DATA_BLOCK "DB_ASI"
TITLE =
VERSION : 0.1


  STRUCT
   SLAVE_1A_IN1 : BOOL ;
   SLAVE_1A_IN2 : BOOL ;
   SLAVE_1A_IN3 : BOOL ;
   SLAVE_1A_IN4 : BOOL ;
   RISERVATO1 : BOOL ;
   RISERVATO2 : BOOL ;
   RISERVATO3 : BOOL ;
   RISERVATO4 : BOOL ;
   SLAVE_3A_IN1 : BOOL ;
   SLAVE_3A_IN2 : BOOL ;
   SLAVE_3A_IN3 : BOOL ;
   SLAVE_3A_IN4 : BOOL ;
   SLAVE_2A_IN1 : BOOL ;
   SLAVE_2A_IN2 : BOOL ;
   SLAVE_2A_IN3 : BOOL ;
   SLAVE_2A_IN4 : BOOL ;
   SLAVE_5A_IN1 : BOOL ;
   SLAVE_5A_IN2 : BOOL ;
   SLAVE_5A_IN3 : BOOL ;
   SLAVE_5A_IN4 : BOOL ;
   SLAVE_4A_IN1 : BOOL ;
   SLAVE_4A_IN2 : BOOL ;
   SLAVE_4A_IN3 : BOOL ;
   SLAVE_4A_IN4 : BOOL ;
   SLAVE_7A_IN1 : BOOL ;
   SLAVE_7A_IN2 : BOOL ;
   SLAVE_7A_IN3 : BOOL ;
   SLAVE_7A_IN4 : BOOL ;
   SLAVE_6A_IN1 : BOOL ;
   SLAVE_6A_IN2 : BOOL ;
   SLAVE_6A_IN3 : BOOL ;
   SLAVE_6A_IN4 : BOOL ;
   SLAVE_9A_IN1 : BOOL ;
   SLAVE_9A_IN2 : BOOL ;
   SLAVE_9A_IN3 : BOOL ;
   SLAVE_9A_IN4 : BOOL ;
   SLAVE_8A_IN1 : BOOL ;
   SLAVE_8A_IN2 : BOOL ;
   SLAVE_8A_IN3 : BOOL ;
   SLAVE_8A_IN4 : BOOL ;
   SLAVE_11A_IN1 : BOOL ;
   SLAVE_11A_IN2 : BOOL ;
   SLAVE_11A_IN3 : BOOL ;
   SLAVE_11A_IN4 : BOOL ;
   SLAVE_10A_IN1 : BOOL ;
   SLAVE_10A_IN2 : BOOL ;
   SLAVE_10A_IN3 : BOOL ;
   SLAVE_10A_IN4 : BOOL ;
   SLAVE_13A_IN1 : BOOL ;
   SLAVE_13A_IN2 : BOOL ;
   SLAVE_13A_IN3 : BOOL ;
   SLAVE_13A_IN4 : BOOL ;
   SLAVE_12A_IN1 : BOOL ;
   SLAVE_12A_IN2 : BOOL ;
   SLAVE_12A_IN3 : BOOL ;
   SLAVE_12A_IN4 : BOOL ;
   SLAVE_15A_IN1 : BOOL ;
   SLAVE_15A_IN2 : BOOL ;
   SLAVE_15A_IN3 : BOOL ;
   SLAVE_15A_IN4 : BOOL ;
   SLAVE_14A_IN1 : BOOL ;
   SLAVE_14A_IN2 : BOOL ;
   SLAVE_14A_IN3 : BOOL ;
   SLAVE_14A_IN4 : BOOL ;
   SLAVE_17A_IN1 : BOOL ;
   SLAVE_17A_IN2 : BOOL ;
   SLAVE_17A_IN3 : BOOL ;
   SLAVE_17A_IN4 : BOOL ;
   SLAVE_16A_IN1 : BOOL ;
   SLAVE_16A_IN2 : BOOL ;
   SLAVE_16A_IN3 : BOOL ;
   SLAVE_16A_IN4 : BOOL ;
   SLAVE_19A_IN1 : BOOL ;
   SLAVE_19A_IN2 : BOOL ;
   SLAVE_19A_IN3 : BOOL ;
   SLAVE_19A_IN4 : BOOL ;
   SLAVE_18A_IN1 : BOOL ;
   SLAVE_18A_IN2 : BOOL ;
   SLAVE_18A_IN3 : BOOL ;
   SLAVE_18A_IN4 : BOOL ;
   SLAVE_21A_IN1 : BOOL ;
   SLAVE_21A_IN2 : BOOL ;
   SLAVE_21A_IN3 : BOOL ;
   SLAVE_21A_IN4 : BOOL ;
   SLAVE_20A_IN1 : BOOL ;
   SLAVE_20A_IN2 : BOOL ;
   SLAVE_20A_IN3 : BOOL ;
   SLAVE_20A_IN4 : BOOL ;
   SLAVE_23A_IN1 : BOOL ;
   SLAVE_23A_IN2 : BOOL ;
   SLAVE_23A_IN3 : BOOL ;
   SLAVE_23A_IN4 : BOOL ;
   SLAVE_22A_IN1 : BOOL ;
   SLAVE_22A_IN2 : BOOL ;
   SLAVE_22A_IN3 : BOOL ;
   SLAVE_22A_IN4 : BOOL ;
   SLAVE_25A_IN1 : BOOL ;
   SLAVE_25A_IN2 : BOOL ;
   SLAVE_25A_IN3 : BOOL ;
   SLAVE_25A_IN4 : BOOL ;
   SLAVE_24A_IN1 : BOOL ;
   SLAVE_24A_IN2 : BOOL ;
   SLAVE_24A_IN3 : BOOL ;
   SLAVE_24A_IN4 : BOOL ;
   SLAVE_27A_IN1 : BOOL ;
   SLAVE_27A_IN2 : BOOL ;
   SLAVE_27A_IN3 : BOOL ;
   SLAVE_27A_IN4 : BOOL ;
   SLAVE_26A_IN1 : BOOL ;
   SLAVE_26A_IN2 : BOOL ;
   SLAVE_26A_IN3 : BOOL ;
   SLAVE_26A_IN4 : BOOL ;
   SLAVE_29A_IN1 : BOOL ;
   SLAVE_29A_IN2 : BOOL ;
   SLAVE_29A_IN3 : BOOL ;
   SLAVE_29A_IN4 : BOOL ;
   SLAVE_28A_IN1 : BOOL ;
   SLAVE_28A_IN2 : BOOL ;
   SLAVE_28A_IN3 : BOOL ;
   SLAVE_28A_IN4 : BOOL ;
   SLAVE_31A_IN1 : BOOL ;
   SLAVE_31A_IN2 : BOOL ;
   SLAVE_31A_IN3 : BOOL ;
   SLAVE_31A_IN4 : BOOL ;
   SLAVE_30A_IN1 : BOOL ;
   SLAVE_30A_IN2 : BOOL ;
   SLAVE_30A_IN3 : BOOL ;
   SLAVE_30A_IN4 : BOOL ;
   SLAVE_1B_IN1 : BOOL ;
   SLAVE_1B_IN2 : BOOL ;
   SLAVE_1B_IN3 : BOOL ;
   SLAVE_1B_IN4 : BOOL ;
   RISERVATO5 : BOOL ;
   RISERVATO6 : BOOL ;
   RISERVATO7 : BOOL ;
   RISERVATO8 : BOOL ;
   SLAVE_3B_IN1 : BOOL ;
   SLAVE_3B_IN2 : BOOL ;
   SLAVE_3B_IN3 : BOOL ;
   SLAVE_3B_IN4 : BOOL ;
   SLAVE_2B_IN1 : BOOL ;
   SLAVE_2B_IN2 : BOOL ;
   SLAVE_2B_IN3 : BOOL ;
   SLAVE_2B_IN4 : BOOL ;
   SLAVE_5B_IN1 : BOOL ;
   SLAVE_5B_IN2 : BOOL ;
   SLAVE_5B_IN3 : BOOL ;
   SLAVE_5B_IN4 : BOOL ;
   SLAVE_4B_IN1 : BOOL ;
   SLAVE_4B_IN2 : BOOL ;
   SLAVE_4B_IN3 : BOOL ;
   SLAVE_4B_IN4 : BOOL ;
   SLAVE_7B_IN1 : BOOL ;
   SLAVE_7B_IN2 : BOOL ;
   SLAVE_7B_IN3 : BOOL ;
   SLAVE_7B_IN4 : BOOL ;
   SLAVE_6B_IN1 : BOOL ;
   SLAVE_6B_IN2 : BOOL ;
   SLAVE_6B_IN3 : BOOL ;
   SLAVE_6B_IN4 : BOOL ;
   SLAVE_9B_IN1 : BOOL ;
   SLAVE_9B_IN2 : BOOL ;
   SLAVE_9B_IN3 : BOOL ;
   SLAVE_9B_IN4 : BOOL ;
   SLAVE_8B_IN1 : BOOL ;
   SLAVE_8B_IN2 : BOOL ;
   SLAVE_8B_IN3 : BOOL ;
   SLAVE_8B_IN4 : BOOL ;
   SLAVE_11B_IN1 : BOOL ;
   SLAVE_11B_IN2 : BOOL ;
   SLAVE_11B_IN3 : BOOL ;
   SLAVE_11B_IN4 : BOOL ;
   SLAVE_10B_IN1 : BOOL ;
   SLAVE_10B_IN2 : BOOL ;
   SLAVE_10B_IN3 : BOOL ;
   SLAVE_10B_IN4 : BOOL ;
   SLAVE_13B_IN1 : BOOL ;
   SLAVE_13B_IN2 : BOOL ;
   SLAVE_13B_IN3 : BOOL ;
   SLAVE_13B_IN4 : BOOL ;
   SLAVE_12B_IN1 : BOOL ;
   SLAVE_12B_IN2 : BOOL ;
   SLAVE_12B_IN3 : BOOL ;
   SLAVE_12B_IN4 : BOOL ;
   SLAVE_15B_IN1 : BOOL ;
   SLAVE_15B_IN2 : BOOL ;
   SLAVE_15B_IN3 : BOOL ;
   SLAVE_15B_IN4 : BOOL ;
   SLAVE_14B_IN1 : BOOL ;
   SLAVE_14B_IN2 : BOOL ;
   SLAVE_14B_IN3 : BOOL ;
   SLAVE_14B_IN4 : BOOL ;
   SLAVE_17B_IN1 : BOOL ;
   SLAVE_17B_IN2 : BOOL ;
   SLAVE_17B_IN3 : BOOL ;
   SLAVE_17B_IN4 : BOOL ;
   SLAVE_16B_IN1 : BOOL ;
   SLAVE_16B_IN2 : BOOL ;
   SLAVE_16B_IN3 : BOOL ;
   SLAVE_16B_IN4 : BOOL ;
   SLAVE_19B_IN1 : BOOL ;
   SLAVE_19B_IN2 : BOOL ;
   SLAVE_19B_IN3 : BOOL ;
   SLAVE_19B_IN4 : BOOL ;
   SLAVE_18B_IN1 : BOOL ;
   SLAVE_18B_IN2 : BOOL ;
   SLAVE_18B_IN3 : BOOL ;
   SLAVE_18B_IN4 : BOOL ;
   SLAVE_21B_IN1 : BOOL ;
   SLAVE_21B_IN2 : BOOL ;
   SLAVE_21B_IN3 : BOOL ;
   SLAVE_21B_IN4 : BOOL ;
   SLAVE_20B_IN1 : BOOL ;
   SLAVE_20B_IN2 : BOOL ;
   SLAVE_20B_IN3 : BOOL ;
   SLAVE_20B_IN4 : BOOL ;
   SLAVE_23B_IN1 : BOOL ;
   SLAVE_23B_IN2 : BOOL ;
   SLAVE_23B_IN3 : BOOL ;
   SLAVE_23B_IN4 : BOOL ;
   SLAVE_22B_IN1 : BOOL ;
   SLAVE_22B_IN2 : BOOL ;
   SLAVE_22B_IN3 : BOOL ;
   SLAVE_22B_IN4 : BOOL ;
   SLAVE_25B_IN1 : BOOL ;
   SLAVE_25B_IN2 : BOOL ;
   SLAVE_25B_IN3 : BOOL ;
   SLAVE_25B_IN4 : BOOL ;
   SLAVE_24B_IN1 : BOOL ;
   SLAVE_24B_IN2 : BOOL ;
   SLAVE_24B_IN3 : BOOL ;
   SLAVE_24B_IN4 : BOOL ;
   SLAVE_27B_IN1 : BOOL ;
   SLAVE_27B_IN2 : BOOL ;
   SLAVE_27B_IN3 : BOOL ;
   SLAVE_27B_IN4 : BOOL ;
   SLAVE_26B_IN1 : BOOL ;
   SLAVE_26B_IN2 : BOOL ;
   SLAVE_26B_IN3 : BOOL ;
   SLAVE_26B_IN4 : BOOL ;
   SLAVE_29B_IN1 : BOOL ;
   SLAVE_29B_IN2 : BOOL ;
   SLAVE_29B_IN3 : BOOL ;
   SLAVE_29B_IN4 : BOOL ;
   SLAVE_28B_IN1 : BOOL ;
   SLAVE_28B_IN2 : BOOL ;
   SLAVE_28B_IN3 : BOOL ;
   SLAVE_28B_IN4 : BOOL ;
   SLAVE_31B_IN1 : BOOL ;
   SLAVE_31B_IN2 : BOOL ;
   SLAVE_31B_IN3 : BOOL ;
   SLAVE_31B_IN4 : BOOL ;
   SLAVE_30B_IN1 : BOOL ;
   SLAVE_30B_IN2 : BOOL ;
   SLAVE_30B_IN3 : BOOL ;
   SLAVE_30B_IN4 : BOOL ;
   SLAVE_1A_OUT1 : BOOL ;
   SLAVE_1A_OUT2 : BOOL ;
   SLAVE_1A_OUT3 : BOOL ;
   SLAVE_1A_OUT4 : BOOL ;
   RISERVATO9 : BOOL ;
   RISERVATO10 : BOOL ;
   RISERVATO11 : BOOL ;
   RISERVATO12 : BOOL ;
   SLAVE_3A_OUT1 : BOOL ;
   SLAVE_3A_OUT2 : BOOL ;
   SLAVE_3A_OUT3 : BOOL ;
   SLAVE_3A_OUT4 : BOOL ;
   SLAVE_2A_OUT1 : BOOL ;
   SLAVE_2A_OUT2 : BOOL ;
   SLAVE_2A_OUT3 : BOOL ;
   SLAVE_2A_OUT4 : BOOL ;
   SLAVE_5A_OUT1 : BOOL ;
   SLAVE_5A_OUT2 : BOOL ;
   SLAVE_5A_OUT3 : BOOL ;
   SLAVE_5A_OUT4 : BOOL ;
   SLAVE_4A_OUT1 : BOOL ;
   SLAVE_4A_OUT2 : BOOL ;
   SLAVE_4A_OUT3 : BOOL ;
   SLAVE_4A_OUT4 : BOOL ;
   SLAVE_7A_OUT1 : BOOL ;
   SLAVE_7A_OUT2 : BOOL ;
   SLAVE_7A_OUT3 : BOOL ;
   SLAVE_7A_OUT4 : BOOL ;
   SLAVE_6A_OUT1 : BOOL ;
   SLAVE_6A_OUT2 : BOOL ;
   SLAVE_6A_OUT3 : BOOL ;
   SLAVE_6A_OUT4 : BOOL ;
   SLAVE_9A_OUT1 : BOOL ;
   SLAVE_9A_OUT2 : BOOL ;
   SLAVE_9A_OUT3 : BOOL ;
   SLAVE_9A_OUT4 : BOOL ;
   SLAVE_8A_OUT1 : BOOL ;
   SLAVE_8A_OUT2 : BOOL ;
   SLAVE_8A_OUT3 : BOOL ;
   SLAVE_8A_OUT4 : BOOL ;
   SLAVE_11A_OUT1 : BOOL ;
   SLAVE_11A_OUT2 : BOOL ;
   SLAVE_11A_OUT3 : BOOL ;
   SLAVE_11A_OUT4 : BOOL ;
   SLAVE_10A_OUT1 : BOOL ;
   SLAVE_10A_OUT2 : BOOL ;
   SLAVE_10A_OUT3 : BOOL ;
   SLAVE_10A_OUT4 : BOOL ;
   SLAVE_13A_OUT1 : BOOL ;
   SLAVE_13A_OUT2 : BOOL ;
   SLAVE_13A_OUT3 : BOOL ;
   SLAVE_13A_OUT4 : BOOL ;
   SLAVE_12A_OUT1 : BOOL ;
   SLAVE_12A_OUT2 : BOOL ;
   SLAVE_12A_OUT3 : BOOL ;
   SLAVE_12A_OUT4 : BOOL ;
   SLAVE_15A_OUT1 : BOOL ;
   SLAVE_15A_OUT2 : BOOL ;
   SLAVE_15A_OUT3 : BOOL ;
   SLAVE_15A_OUT4 : BOOL ;
   SLAVE_14A_OUT1 : BOOL ;
   SLAVE_14A_OUT2 : BOOL ;
   SLAVE_14A_OUT3 : BOOL ;
   SLAVE_14A_OUT4 : BOOL ;
   SLAVE_17A_OUT1 : BOOL ;
   SLAVE_17A_OUT2 : BOOL ;
   SLAVE_17A_OUT3 : BOOL ;
   SLAVE_17A_OUT4 : BOOL ;
   SLAVE_16A_OUT1 : BOOL ;
   SLAVE_16A_OUT2 : BOOL ;
   SLAVE_16A_OUT3 : BOOL ;
   SLAVE_16A_OUT4 : BOOL ;
   SLAVE_19A_OUT1 : BOOL ;
   SLAVE_19A_OUT2 : BOOL ;
   SLAVE_19A_OUT3 : BOOL ;
   SLAVE_19A_OUT4 : BOOL ;
   SLAVE_18A_OUT1 : BOOL ;
   SLAVE_18A_OUT2 : BOOL ;
   SLAVE_18A_OUT3 : BOOL ;
   SLAVE_18A_OUT4 : BOOL ;
   SLAVE_21A_OUT1 : BOOL ;
   SLAVE_21A_OUT2 : BOOL ;
   SLAVE_21A_OUT3 : BOOL ;
   SLAVE_21A_OUT4 : BOOL ;
   SLAVE_20A_OUT1 : BOOL ;
   SLAVE_20A_OUT2 : BOOL ;
   SLAVE_20A_OUT3 : BOOL ;
   SLAVE_20A_OUT4 : BOOL ;
   SLAVE_23A_OUT1 : BOOL ;
   SLAVE_23A_OUT2 : BOOL ;
   SLAVE_23A_OUT3 : BOOL ;
   SLAVE_23A_OUT4 : BOOL ;
   SLAVE_22A_OUT1 : BOOL ;
   SLAVE_22A_OUT2 : BOOL ;
   SLAVE_22A_OUT3 : BOOL ;
   SLAVE_22A_OUT4 : BOOL ;
   SLAVE_25A_OUT1 : BOOL ;
   SLAVE_25A_OUT2 : BOOL ;
   SLAVE_25A_OUT3 : BOOL ;
   SLAVE_25A_OUT4 : BOOL ;
   SLAVE_24A_OUT1 : BOOL ;
   SLAVE_24A_OUT2 : BOOL ;
   SLAVE_24A_OUT3 : BOOL ;
   SLAVE_24A_OUT4 : BOOL ;
   SLAVE_27A_OUT1 : BOOL ;
   SLAVE_27A_OUT2 : BOOL ;
   SLAVE_27A_OUT3 : BOOL ;
   SLAVE_27A_OUT4 : BOOL ;
   SLAVE_26A_OUT1 : BOOL ;
   SLAVE_26A_OUT2 : BOOL ;
   SLAVE_26A_OUT3 : BOOL ;
   SLAVE_26A_OUT4 : BOOL ;
   SLAVE_29A_OUT1 : BOOL ;
   SLAVE_29A_OUT2 : BOOL ;
   SLAVE_29A_OUT3 : BOOL ;
   SLAVE_29A_OUT4 : BOOL ;
   SLAVE_28A_OUT1 : BOOL ;
   SLAVE_28A_OUT2 : BOOL ;
   SLAVE_28A_OUT3 : BOOL ;
   SLAVE_28A_OUT4 : BOOL ;
   SLAVE_31A_OUT1 : BOOL ;
   SLAVE_31A_OUT2 : BOOL ;
   SLAVE_31A_OUT3 : BOOL ;
   SLAVE_31A_OUT4 : BOOL ;
   SLAVE_30A_OUT1 : BOOL ;
   SLAVE_30A_OUT2 : BOOL ;
   SLAVE_30A_OUT3 : BOOL ;
   SLAVE_30A_OUT4 : BOOL ;
   SLAVE_1B_OUT1 : BOOL ;
   SLAVE_1B_OUT2 : BOOL ;
   SLAVE_1B_OUT3 : BOOL ;
   SLAVE_1B_OUT4 : BOOL ;
   RISERVATO13 : BOOL ;
   RISERVATO14 : BOOL ;
   RISERVATO15 : BOOL ;
   RISERVATO16 : BOOL ;
   SLAVE_3B_OUT1 : BOOL ;
   SLAVE_3B_OUT2 : BOOL ;
   SLAVE_3B_OUT3 : BOOL ;
   SLAVE_3B_OUT4 : BOOL ;
   SLAVE_2B_OUT1 : BOOL ;
   SLAVE_2B_OUT2 : BOOL ;
   SLAVE_2B_OUT3 : BOOL ;
   SLAVE_2B_OUT4 : BOOL ;
   SLAVE_5B_OUT1 : BOOL ;
   SLAVE_5B_OUT2 : BOOL ;
   SLAVE_5B_OUT3 : BOOL ;
   SLAVE_5B_OUT4 : BOOL ;
   SLAVE_4B_OUT1 : BOOL ;
   SLAVE_4B_OUT2 : BOOL ;
   SLAVE_4B_OUT3 : BOOL ;
   SLAVE_4B_OUT4 : BOOL ;
   SLAVE_7B_OUT1 : BOOL ;
   SLAVE_7B_OUT2 : BOOL ;
   SLAVE_7B_OUT3 : BOOL ;
   SLAVE_7B_OUT4 : BOOL ;
   SLAVE_6B_OUT1 : BOOL ;
   SLAVE_6B_OUT2 : BOOL ;
   SLAVE_6B_OUT3 : BOOL ;
   SLAVE_6B_OUT4 : BOOL ;
   SLAVE_9B_OUT1 : BOOL ;
   SLAVE_9B_OUT2 : BOOL ;
   SLAVE_9B_OUT3 : BOOL ;
   SLAVE_9B_OUT4 : BOOL ;
   SLAVE_8B_OUT1 : BOOL ;
   SLAVE_8B_OUT2 : BOOL ;
   SLAVE_8B_OUT3 : BOOL ;
   SLAVE_8B_OUT4 : BOOL ;
   SLAVE_11B_OUT1 : BOOL ;
   SLAVE_11B_OUT2 : BOOL ;
   SLAVE_11B_OUT3 : BOOL ;
   SLAVE_11B_OUT4 : BOOL ;
   SLAVE_10B_OUT1 : BOOL ;
   SLAVE_10B_OUT2 : BOOL ;
   SLAVE_10B_OUT3 : BOOL ;
   SLAVE_10B_OUT4 : BOOL ;
   SLAVE_13B_OUT1 : BOOL ;
   SLAVE_13B_OUT2 : BOOL ;
   SLAVE_13B_OUT3 : BOOL ;
   SLAVE_13B_OUT4 : BOOL ;
   SLAVE_12B_OUT1 : BOOL ;
   SLAVE_12B_OUT2 : BOOL ;
   SLAVE_12B_OUT3 : BOOL ;
   SLAVE_12B_OUT4 : BOOL ;
   SLAVE_15B_OUT1 : BOOL ;
   SLAVE_15B_OUT2 : BOOL ;
   SLAVE_15B_OUT3 : BOOL ;
   SLAVE_15B_OUT4 : BOOL ;
   SLAVE_14B_OUT1 : BOOL ;
   SLAVE_14B_OUT2 : BOOL ;
   SLAVE_14B_OUT3 : BOOL ;
   SLAVE_14B_OUT4 : BOOL ;
   SLAVE_17B_OUT1 : BOOL ;
   SLAVE_17B_OUT2 : BOOL ;
   SLAVE_17B_OUT3 : BOOL ;
   SLAVE_17B_OUT4 : BOOL ;
   SLAVE_16B_OUT1 : BOOL ;
   SLAVE_16B_OUT2 : BOOL ;
   SLAVE_16B_OUT3 : BOOL ;
   SLAVE_16B_OUT4 : BOOL ;
   SLAVE_19B_OUT1 : BOOL ;
   SLAVE_19B_OUT2 : BOOL ;
   SLAVE_19B_OUT3 : BOOL ;
   SLAVE_19B_OUT4 : BOOL ;
   SLAVE_18B_OUT1 : BOOL ;
   SLAVE_18B_OUT2 : BOOL ;
   SLAVE_18B_OUT3 : BOOL ;
   SLAVE_18B_OUT4 : BOOL ;
   SLAVE_21B_OUT1 : BOOL ;
   SLAVE_21B_OUT2 : BOOL ;
   SLAVE_21B_OUT3 : BOOL ;
   SLAVE_21B_OUT4 : BOOL ;
   SLAVE_20B_OUT1 : BOOL ;
   SLAVE_20B_OUT2 : BOOL ;
   SLAVE_20B_OUT3 : BOOL ;
   SLAVE_20B_OUT4 : BOOL ;
   SLAVE_23B_OUT1 : BOOL ;
   SLAVE_23B_OUT2 : BOOL ;
   SLAVE_23B_OUT3 : BOOL ;
   SLAVE_23B_OUT4 : BOOL ;
   SLAVE_22B_OUT1 : BOOL ;
   SLAVE_22B_OUT2 : BOOL ;
   SLAVE_22B_OUT3 : BOOL ;
   SLAVE_22B_OUT4 : BOOL ;
   SLAVE_25B_OUT1 : BOOL ;
   SLAVE_25B_OUT2 : BOOL ;
   SLAVE_25B_OUT3 : BOOL ;
   SLAVE_25B_OUT4 : BOOL ;
   SLAVE_24B_OUT1 : BOOL ;
   SLAVE_24B_OUT2 : BOOL ;
   SLAVE_24B_OUT3 : BOOL ;
   SLAVE_24B_OUT4 : BOOL ;
   SLAVE_27B_OUT1 : BOOL ;
   SLAVE_27B_OUT2 : BOOL ;
   SLAVE_27B_OUT3 : BOOL ;
   SLAVE_27B_OUT4 : BOOL ;
   SLAVE_26B_OUT1 : BOOL ;
   SLAVE_26B_OUT2 : BOOL ;
   SLAVE_26B_OUT3 : BOOL ;
   SLAVE_26B_OUT4 : BOOL ;
   SLAVE_29B_OUT1 : BOOL ;
   SLAVE_29B_OUT2 : BOOL ;
   SLAVE_29B_OUT3 : BOOL ;
   SLAVE_29B_OUT4 : BOOL ;
   SLAVE_28B_OUT1 : BOOL ;
   SLAVE_28B_OUT2 : BOOL ;
   SLAVE_28B_OUT3 : BOOL ;
   SLAVE_28B_OUT4 : BOOL ;
   SLAVE_31B_OUT1 : BOOL ;
   SLAVE_31B_OUT2 : BOOL ;
   SLAVE_31B_OUT3 : BOOL ;
   SLAVE_31B_OUT4 : BOOL ;
   SLAVE_30B_OUT1 : BOOL ;
   SLAVE_30B_OUT2 : BOOL ;
   SLAVE_30B_OUT3 : BOOL ;
   SLAVE_30B_OUT4 : BOOL ;
  END_STRUCT ;
BEGIN
   SLAVE_1A_IN1 := FALSE;
   SLAVE_1A_IN2 := FALSE;
   SLAVE_1A_IN3 := FALSE;
   SLAVE_1A_IN4 := FALSE;
   RISERVATO1 := FALSE;
   RISERVATO2 := FALSE;
   RISERVATO3 := FALSE;
   RISERVATO4 := FALSE;
   SLAVE_3A_IN1 := FALSE;
   SLAVE_3A_IN2 := FALSE;
   SLAVE_3A_IN3 := FALSE;
   SLAVE_3A_IN4 := FALSE;
   SLAVE_2A_IN1 := FALSE;
   SLAVE_2A_IN2 := FALSE;
   SLAVE_2A_IN3 := FALSE;
   SLAVE_2A_IN4 := FALSE;
   SLAVE_5A_IN1 := FALSE;
   SLAVE_5A_IN2 := FALSE;
   SLAVE_5A_IN3 := FALSE;
   SLAVE_5A_IN4 := FALSE;
   SLAVE_4A_IN1 := FALSE;
   SLAVE_4A_IN2 := FALSE;
   SLAVE_4A_IN3 := FALSE;
   SLAVE_4A_IN4 := FALSE;
   SLAVE_7A_IN1 := FALSE;
   SLAVE_7A_IN2 := FALSE;
   SLAVE_7A_IN3 := FALSE;
   SLAVE_7A_IN4 := FALSE;
   SLAVE_6A_IN1 := FALSE;
   SLAVE_6A_IN2 := FALSE;
   SLAVE_6A_IN3 := FALSE;
   SLAVE_6A_IN4 := FALSE;
   SLAVE_9A_IN1 := FALSE;
   SLAVE_9A_IN2 := FALSE;
   SLAVE_9A_IN3 := FALSE;
   SLAVE_9A_IN4 := FALSE;
   SLAVE_8A_IN1 := FALSE;
   SLAVE_8A_IN2 := FALSE;
   SLAVE_8A_IN3 := FALSE;
   SLAVE_8A_IN4 := FALSE;
   SLAVE_11A_IN1 := FALSE;
   SLAVE_11A_IN2 := FALSE;
   SLAVE_11A_IN3 := FALSE;
   SLAVE_11A_IN4 := FALSE;
   SLAVE_10A_IN1 := FALSE;
   SLAVE_10A_IN2 := FALSE;
   SLAVE_10A_IN3 := FALSE;
   SLAVE_10A_IN4 := FALSE;
   SLAVE_13A_IN1 := FALSE;
   SLAVE_13A_IN2 := FALSE;
   SLAVE_13A_IN3 := FALSE;
   SLAVE_13A_IN4 := FALSE;
   SLAVE_12A_IN1 := FALSE;
   SLAVE_12A_IN2 := FALSE;
   SLAVE_12A_IN3 := FALSE;
   SLAVE_12A_IN4 := FALSE;
   SLAVE_15A_IN1 := FALSE;
   SLAVE_15A_IN2 := FALSE;
   SLAVE_15A_IN3 := FALSE;
   SLAVE_15A_IN4 := FALSE;
   SLAVE_14A_IN1 := FALSE;
   SLAVE_14A_IN2 := FALSE;
   SLAVE_14A_IN3 := FALSE;
   SLAVE_14A_IN4 := FALSE;
   SLAVE_17A_IN1 := FALSE;
   SLAVE_17A_IN2 := FALSE;
   SLAVE_17A_IN3 := FALSE;
   SLAVE_17A_IN4 := FALSE;
   SLAVE_16A_IN1 := FALSE;
   SLAVE_16A_IN2 := FALSE;
   SLAVE_16A_IN3 := FALSE;
   SLAVE_16A_IN4 := FALSE;
   SLAVE_19A_IN1 := FALSE;
   SLAVE_19A_IN2 := FALSE;
   SLAVE_19A_IN3 := FALSE;
   SLAVE_19A_IN4 := FALSE;
   SLAVE_18A_IN1 := FALSE;
   SLAVE_18A_IN2 := FALSE;
   SLAVE_18A_IN3 := FALSE;
   SLAVE_18A_IN4 := FALSE;
   SLAVE_21A_IN1 := FALSE;
   SLAVE_21A_IN2 := FALSE;
   SLAVE_21A_IN3 := FALSE;
   SLAVE_21A_IN4 := FALSE;
   SLAVE_20A_IN1 := FALSE;
   SLAVE_20A_IN2 := FALSE;
   SLAVE_20A_IN3 := FALSE;
   SLAVE_20A_IN4 := FALSE;
   SLAVE_23A_IN1 := FALSE;
   SLAVE_23A_IN2 := FALSE;
   SLAVE_23A_IN3 := FALSE;
   SLAVE_23A_IN4 := FALSE;
   SLAVE_22A_IN1 := FALSE;
   SLAVE_22A_IN2 := FALSE;
   SLAVE_22A_IN3 := FALSE;
   SLAVE_22A_IN4 := FALSE;
   SLAVE_25A_IN1 := FALSE;
   SLAVE_25A_IN2 := FALSE;
   SLAVE_25A_IN3 := FALSE;
   SLAVE_25A_IN4 := FALSE;
   SLAVE_24A_IN1 := FALSE;
   SLAVE_24A_IN2 := FALSE;
   SLAVE_24A_IN3 := FALSE;
   SLAVE_24A_IN4 := FALSE;
   SLAVE_27A_IN1 := FALSE;
   SLAVE_27A_IN2 := FALSE;
   SLAVE_27A_IN3 := FALSE;
   SLAVE_27A_IN4 := FALSE;
   SLAVE_26A_IN1 := FALSE;
   SLAVE_26A_IN2 := FALSE;
   SLAVE_26A_IN3 := FALSE;
   SLAVE_26A_IN4 := FALSE;
   SLAVE_29A_IN1 := FALSE;
   SLAVE_29A_IN2 := FALSE;
   SLAVE_29A_IN3 := FALSE;
   SLAVE_29A_IN4 := FALSE;
   SLAVE_28A_IN1 := FALSE;
   SLAVE_28A_IN2 := FALSE;
   SLAVE_28A_IN3 := FALSE;
   SLAVE_28A_IN4 := FALSE;
   SLAVE_31A_IN1 := FALSE;
   SLAVE_31A_IN2 := FALSE;
   SLAVE_31A_IN3 := FALSE;
   SLAVE_31A_IN4 := FALSE;
   SLAVE_30A_IN1 := FALSE;
   SLAVE_30A_IN2 := FALSE;
   SLAVE_30A_IN3 := FALSE;
   SLAVE_30A_IN4 := FALSE;
   SLAVE_1B_IN1 := FALSE;
   SLAVE_1B_IN2 := FALSE;
   SLAVE_1B_IN3 := FALSE;
   SLAVE_1B_IN4 := FALSE;
   RISERVATO5 := FALSE;
   RISERVATO6 := FALSE;
   RISERVATO7 := FALSE;
   RISERVATO8 := FALSE;
   SLAVE_3B_IN1 := FALSE;
   SLAVE_3B_IN2 := FALSE;
   SLAVE_3B_IN3 := FALSE;
   SLAVE_3B_IN4 := FALSE;
   SLAVE_2B_IN1 := FALSE;
   SLAVE_2B_IN2 := FALSE;
   SLAVE_2B_IN3 := FALSE;
   SLAVE_2B_IN4 := FALSE;
   SLAVE_5B_IN1 := FALSE;
   SLAVE_5B_IN2 := FALSE;
   SLAVE_5B_IN3 := FALSE;
   SLAVE_5B_IN4 := FALSE;
   SLAVE_4B_IN1 := FALSE;
   SLAVE_4B_IN2 := FALSE;
   SLAVE_4B_IN3 := FALSE;
   SLAVE_4B_IN4 := FALSE;
   SLAVE_7B_IN1 := FALSE;
   SLAVE_7B_IN2 := FALSE;
   SLAVE_7B_IN3 := FALSE;
   SLAVE_7B_IN4 := FALSE;
   SLAVE_6B_IN1 := FALSE;
   SLAVE_6B_IN2 := FALSE;
   SLAVE_6B_IN3 := FALSE;
   SLAVE_6B_IN4 := FALSE;
   SLAVE_9B_IN1 := FALSE;
   SLAVE_9B_IN2 := FALSE;
   SLAVE_9B_IN3 := FALSE;
   SLAVE_9B_IN4 := FALSE;
   SLAVE_8B_IN1 := FALSE;
   SLAVE_8B_IN2 := FALSE;
   SLAVE_8B_IN3 := FALSE;
   SLAVE_8B_IN4 := FALSE;
   SLAVE_11B_IN1 := FALSE;
   SLAVE_11B_IN2 := FALSE;
   SLAVE_11B_IN3 := FALSE;
   SLAVE_11B_IN4 := FALSE;
   SLAVE_10B_IN1 := FALSE;
   SLAVE_10B_IN2 := FALSE;
   SLAVE_10B_IN3 := FALSE;
   SLAVE_10B_IN4 := FALSE;
   SLAVE_13B_IN1 := FALSE;
   SLAVE_13B_IN2 := FALSE;
   SLAVE_13B_IN3 := FALSE;
   SLAVE_13B_IN4 := FALSE;
   SLAVE_12B_IN1 := FALSE;
   SLAVE_12B_IN2 := FALSE;
   SLAVE_12B_IN3 := FALSE;
   SLAVE_12B_IN4 := FALSE;
   SLAVE_15B_IN1 := FALSE;
   SLAVE_15B_IN2 := FALSE;
   SLAVE_15B_IN3 := FALSE;
   SLAVE_15B_IN4 := FALSE;
   SLAVE_14B_IN1 := FALSE;
   SLAVE_14B_IN2 := FALSE;
   SLAVE_14B_IN3 := FALSE;
   SLAVE_14B_IN4 := FALSE;
   SLAVE_17B_IN1 := FALSE;
   SLAVE_17B_IN2 := FALSE;
   SLAVE_17B_IN3 := FALSE;
   SLAVE_17B_IN4 := FALSE;
   SLAVE_16B_IN1 := FALSE;
   SLAVE_16B_IN2 := FALSE;
   SLAVE_16B_IN3 := FALSE;
   SLAVE_16B_IN4 := FALSE;
   SLAVE_19B_IN1 := FALSE;
   SLAVE_19B_IN2 := FALSE;
   SLAVE_19B_IN3 := FALSE;
   SLAVE_19B_IN4 := FALSE;
   SLAVE_18B_IN1 := FALSE;
   SLAVE_18B_IN2 := FALSE;
   SLAVE_18B_IN3 := FALSE;
   SLAVE_18B_IN4 := FALSE;
   SLAVE_21B_IN1 := FALSE;
   SLAVE_21B_IN2 := FALSE;
   SLAVE_21B_IN3 := FALSE;
   SLAVE_21B_IN4 := FALSE;
   SLAVE_20B_IN1 := FALSE;
   SLAVE_20B_IN2 := FALSE;
   SLAVE_20B_IN3 := FALSE;
   SLAVE_20B_IN4 := FALSE;
   SLAVE_23B_IN1 := FALSE;
   SLAVE_23B_IN2 := FALSE;
   SLAVE_23B_IN3 := FALSE;
   SLAVE_23B_IN4 := FALSE;
   SLAVE_22B_IN1 := FALSE;
   SLAVE_22B_IN2 := FALSE;
   SLAVE_22B_IN3 := FALSE;
   SLAVE_22B_IN4 := FALSE;
   SLAVE_25B_IN1 := FALSE;
   SLAVE_25B_IN2 := FALSE;
   SLAVE_25B_IN3 := FALSE;
   SLAVE_25B_IN4 := FALSE;
   SLAVE_24B_IN1 := FALSE;
   SLAVE_24B_IN2 := FALSE;
   SLAVE_24B_IN3 := FALSE;
   SLAVE_24B_IN4 := FALSE;
   SLAVE_27B_IN1 := FALSE;
   SLAVE_27B_IN2 := FALSE;
   SLAVE_27B_IN3 := FALSE;
   SLAVE_27B_IN4 := FALSE;
   SLAVE_26B_IN1 := FALSE;
   SLAVE_26B_IN2 := FALSE;
   SLAVE_26B_IN3 := FALSE;
   SLAVE_26B_IN4 := FALSE;
   SLAVE_29B_IN1 := FALSE;
   SLAVE_29B_IN2 := FALSE;
   SLAVE_29B_IN3 := FALSE;
   SLAVE_29B_IN4 := FALSE;
   SLAVE_28B_IN1 := FALSE;
   SLAVE_28B_IN2 := FALSE;
   SLAVE_28B_IN3 := FALSE;
   SLAVE_28B_IN4 := FALSE;
   SLAVE_31B_IN1 := FALSE;
   SLAVE_31B_IN2 := FALSE;
   SLAVE_31B_IN3 := FALSE;
   SLAVE_31B_IN4 := FALSE;
   SLAVE_30B_IN1 := FALSE;
   SLAVE_30B_IN2 := FALSE;
   SLAVE_30B_IN3 := FALSE;
   SLAVE_30B_IN4 := FALSE;
   SLAVE_1A_OUT1 := FALSE;
   SLAVE_1A_OUT2 := FALSE;
   SLAVE_1A_OUT3 := FALSE;
   SLAVE_1A_OUT4 := FALSE;
   RISERVATO9 := FALSE;
   RISERVATO10 := FALSE;
   RISERVATO11 := FALSE;
   RISERVATO12 := FALSE;
   SLAVE_3A_OUT1 := FALSE;
   SLAVE_3A_OUT2 := FALSE;
   SLAVE_3A_OUT3 := FALSE;
   SLAVE_3A_OUT4 := FALSE;
   SLAVE_2A_OUT1 := FALSE;
   SLAVE_2A_OUT2 := FALSE;
   SLAVE_2A_OUT3 := FALSE;
   SLAVE_2A_OUT4 := FALSE;
   SLAVE_5A_OUT1 := FALSE;
   SLAVE_5A_OUT2 := FALSE;
   SLAVE_5A_OUT3 := FALSE;
   SLAVE_5A_OUT4 := FALSE;
   SLAVE_4A_OUT1 := FALSE;
   SLAVE_4A_OUT2 := FALSE;
   SLAVE_4A_OUT3 := FALSE;
   SLAVE_4A_OUT4 := FALSE;
   SLAVE_7A_OUT1 := FALSE;
   SLAVE_7A_OUT2 := FALSE;
   SLAVE_7A_OUT3 := FALSE;
   SLAVE_7A_OUT4 := FALSE;
   SLAVE_6A_OUT1 := FALSE;
   SLAVE_6A_OUT2 := FALSE;
   SLAVE_6A_OUT3 := FALSE;
   SLAVE_6A_OUT4 := FALSE;
   SLAVE_9A_OUT1 := FALSE;
   SLAVE_9A_OUT2 := FALSE;
   SLAVE_9A_OUT3 := FALSE;
   SLAVE_9A_OUT4 := FALSE;
   SLAVE_8A_OUT1 := FALSE;
   SLAVE_8A_OUT2 := FALSE;
   SLAVE_8A_OUT3 := FALSE;
   SLAVE_8A_OUT4 := FALSE;
   SLAVE_11A_OUT1 := FALSE;
   SLAVE_11A_OUT2 := FALSE;
   SLAVE_11A_OUT3 := FALSE;
   SLAVE_11A_OUT4 := FALSE;
   SLAVE_10A_OUT1 := FALSE;
   SLAVE_10A_OUT2 := FALSE;
   SLAVE_10A_OUT3 := FALSE;
   SLAVE_10A_OUT4 := FALSE;
   SLAVE_13A_OUT1 := FALSE;
   SLAVE_13A_OUT2 := FALSE;
   SLAVE_13A_OUT3 := FALSE;
   SLAVE_13A_OUT4 := FALSE;
   SLAVE_12A_OUT1 := FALSE;
   SLAVE_12A_OUT2 := FALSE;
   SLAVE_12A_OUT3 := FALSE;
   SLAVE_12A_OUT4 := FALSE;
   SLAVE_15A_OUT1 := FALSE;
   SLAVE_15A_OUT2 := FALSE;
   SLAVE_15A_OUT3 := FALSE;
   SLAVE_15A_OUT4 := FALSE;
   SLAVE_14A_OUT1 := FALSE;
   SLAVE_14A_OUT2 := FALSE;
   SLAVE_14A_OUT3 := FALSE;
   SLAVE_14A_OUT4 := FALSE;
   SLAVE_17A_OUT1 := FALSE;
   SLAVE_17A_OUT2 := FALSE;
   SLAVE_17A_OUT3 := FALSE;
   SLAVE_17A_OUT4 := FALSE;
   SLAVE_16A_OUT1 := FALSE;
   SLAVE_16A_OUT2 := FALSE;
   SLAVE_16A_OUT3 := FALSE;
   SLAVE_16A_OUT4 := FALSE;
   SLAVE_19A_OUT1 := FALSE;
   SLAVE_19A_OUT2 := FALSE;
   SLAVE_19A_OUT3 := FALSE;
   SLAVE_19A_OUT4 := FALSE;
   SLAVE_18A_OUT1 := FALSE;
   SLAVE_18A_OUT2 := FALSE;
   SLAVE_18A_OUT3 := FALSE;
   SLAVE_18A_OUT4 := FALSE;
   SLAVE_21A_OUT1 := FALSE;
   SLAVE_21A_OUT2 := FALSE;
   SLAVE_21A_OUT3 := FALSE;
   SLAVE_21A_OUT4 := FALSE;
   SLAVE_20A_OUT1 := FALSE;
   SLAVE_20A_OUT2 := FALSE;
   SLAVE_20A_OUT3 := FALSE;
   SLAVE_20A_OUT4 := FALSE;
   SLAVE_23A_OUT1 := FALSE;
   SLAVE_23A_OUT2 := FALSE;
   SLAVE_23A_OUT3 := FALSE;
   SLAVE_23A_OUT4 := FALSE;
   SLAVE_22A_OUT1 := FALSE;
   SLAVE_22A_OUT2 := FALSE;
   SLAVE_22A_OUT3 := FALSE;
   SLAVE_22A_OUT4 := FALSE;
   SLAVE_25A_OUT1 := FALSE;
   SLAVE_25A_OUT2 := FALSE;
   SLAVE_25A_OUT3 := FALSE;
   SLAVE_25A_OUT4 := FALSE;
   SLAVE_24A_OUT1 := FALSE;
   SLAVE_24A_OUT2 := FALSE;
   SLAVE_24A_OUT3 := FALSE;
   SLAVE_24A_OUT4 := FALSE;
   SLAVE_27A_OUT1 := FALSE;
   SLAVE_27A_OUT2 := FALSE;
   SLAVE_27A_OUT3 := FALSE;
   SLAVE_27A_OUT4 := FALSE;
   SLAVE_26A_OUT1 := FALSE;
   SLAVE_26A_OUT2 := FALSE;
   SLAVE_26A_OUT3 := FALSE;
   SLAVE_26A_OUT4 := FALSE;
   SLAVE_29A_OUT1 := FALSE;
   SLAVE_29A_OUT2 := FALSE;
   SLAVE_29A_OUT3 := FALSE;
   SLAVE_29A_OUT4 := FALSE;
   SLAVE_28A_OUT1 := FALSE;
   SLAVE_28A_OUT2 := FALSE;
   SLAVE_28A_OUT3 := FALSE;
   SLAVE_28A_OUT4 := FALSE;
   SLAVE_31A_OUT1 := FALSE;
   SLAVE_31A_OUT2 := FALSE;
   SLAVE_31A_OUT3 := FALSE;
   SLAVE_31A_OUT4 := FALSE;
   SLAVE_30A_OUT1 := FALSE;
   SLAVE_30A_OUT2 := FALSE;
   SLAVE_30A_OUT3 := FALSE;
   SLAVE_30A_OUT4 := FALSE;
   SLAVE_1B_OUT1 := FALSE;
   SLAVE_1B_OUT2 := FALSE;
   SLAVE_1B_OUT3 := FALSE;
   SLAVE_1B_OUT4 := FALSE;
   RISERVATO13 := FALSE;
   RISERVATO14 := FALSE;
   RISERVATO15 := FALSE;
   RISERVATO16 := FALSE;
   SLAVE_3B_OUT1 := FALSE;
   SLAVE_3B_OUT2 := FALSE;
   SLAVE_3B_OUT3 := FALSE;
   SLAVE_3B_OUT4 := FALSE;
   SLAVE_2B_OUT1 := FALSE;
   SLAVE_2B_OUT2 := FALSE;
   SLAVE_2B_OUT3 := FALSE;
   SLAVE_2B_OUT4 := FALSE;
   SLAVE_5B_OUT1 := FALSE;
   SLAVE_5B_OUT2 := FALSE;
   SLAVE_5B_OUT3 := FALSE;
   SLAVE_5B_OUT4 := FALSE;
   SLAVE_4B_OUT1 := FALSE;
   SLAVE_4B_OUT2 := FALSE;
   SLAVE_4B_OUT3 := FALSE;
   SLAVE_4B_OUT4 := FALSE;
   SLAVE_7B_OUT1 := FALSE;
   SLAVE_7B_OUT2 := FALSE;
   SLAVE_7B_OUT3 := FALSE;
   SLAVE_7B_OUT4 := FALSE;
   SLAVE_6B_OUT1 := FALSE;
   SLAVE_6B_OUT2 := FALSE;
   SLAVE_6B_OUT3 := FALSE;
   SLAVE_6B_OUT4 := FALSE;
   SLAVE_9B_OUT1 := FALSE;
   SLAVE_9B_OUT2 := FALSE;
   SLAVE_9B_OUT3 := FALSE;
   SLAVE_9B_OUT4 := FALSE;
   SLAVE_8B_OUT1 := FALSE;
   SLAVE_8B_OUT2 := FALSE;
   SLAVE_8B_OUT3 := FALSE;
   SLAVE_8B_OUT4 := FALSE;
   SLAVE_11B_OUT1 := FALSE;
   SLAVE_11B_OUT2 := FALSE;
   SLAVE_11B_OUT3 := FALSE;
   SLAVE_11B_OUT4 := FALSE;
   SLAVE_10B_OUT1 := FALSE;
   SLAVE_10B_OUT2 := FALSE;
   SLAVE_10B_OUT3 := FALSE;
   SLAVE_10B_OUT4 := FALSE;
   SLAVE_13B_OUT1 := FALSE;
   SLAVE_13B_OUT2 := FALSE;
   SLAVE_13B_OUT3 := FALSE;
   SLAVE_13B_OUT4 := FALSE;
   SLAVE_12B_OUT1 := FALSE;
   SLAVE_12B_OUT2 := FALSE;
   SLAVE_12B_OUT3 := FALSE;
   SLAVE_12B_OUT4 := FALSE;
   SLAVE_15B_OUT1 := FALSE;
   SLAVE_15B_OUT2 := FALSE;
   SLAVE_15B_OUT3 := FALSE;
   SLAVE_15B_OUT4 := FALSE;
   SLAVE_14B_OUT1 := FALSE;
   SLAVE_14B_OUT2 := FALSE;
   SLAVE_14B_OUT3 := FALSE;
   SLAVE_14B_OUT4 := FALSE;
   SLAVE_17B_OUT1 := FALSE;
   SLAVE_17B_OUT2 := FALSE;
   SLAVE_17B_OUT3 := FALSE;
   SLAVE_17B_OUT4 := FALSE;
   SLAVE_16B_OUT1 := FALSE;
   SLAVE_16B_OUT2 := FALSE;
   SLAVE_16B_OUT3 := FALSE;
   SLAVE_16B_OUT4 := FALSE;
   SLAVE_19B_OUT1 := FALSE;
   SLAVE_19B_OUT2 := FALSE;
   SLAVE_19B_OUT3 := FALSE;
   SLAVE_19B_OUT4 := FALSE;
   SLAVE_18B_OUT1 := FALSE;
   SLAVE_18B_OUT2 := FALSE;
   SLAVE_18B_OUT3 := FALSE;
   SLAVE_18B_OUT4 := FALSE;
   SLAVE_21B_OUT1 := FALSE;
   SLAVE_21B_OUT2 := FALSE;
   SLAVE_21B_OUT3 := FALSE;
   SLAVE_21B_OUT4 := FALSE;
   SLAVE_20B_OUT1 := FALSE;
   SLAVE_20B_OUT2 := FALSE;
   SLAVE_20B_OUT3 := FALSE;
   SLAVE_20B_OUT4 := FALSE;
   SLAVE_23B_OUT1 := FALSE;
   SLAVE_23B_OUT2 := FALSE;
   SLAVE_23B_OUT3 := FALSE;
   SLAVE_23B_OUT4 := FALSE;
   SLAVE_22B_OUT1 := FALSE;
   SLAVE_22B_OUT2 := FALSE;
   SLAVE_22B_OUT3 := FALSE;
   SLAVE_22B_OUT4 := FALSE;
   SLAVE_25B_OUT1 := FALSE;
   SLAVE_25B_OUT2 := FALSE;
   SLAVE_25B_OUT3 := FALSE;
   SLAVE_25B_OUT4 := FALSE;
   SLAVE_24B_OUT1 := FALSE;
   SLAVE_24B_OUT2 := FALSE;
   SLAVE_24B_OUT3 := FALSE;
   SLAVE_24B_OUT4 := FALSE;
   SLAVE_27B_OUT1 := FALSE;
   SLAVE_27B_OUT2 := FALSE;
   SLAVE_27B_OUT3 := FALSE;
   SLAVE_27B_OUT4 := FALSE;
   SLAVE_26B_OUT1 := FALSE;
   SLAVE_26B_OUT2 := FALSE;
   SLAVE_26B_OUT3 := FALSE;
   SLAVE_26B_OUT4 := FALSE;
   SLAVE_29B_OUT1 := FALSE;
   SLAVE_29B_OUT2 := FALSE;
   SLAVE_29B_OUT3 := FALSE;
   SLAVE_29B_OUT4 := FALSE;
   SLAVE_28B_OUT1 := FALSE;
   SLAVE_28B_OUT2 := FALSE;
   SLAVE_28B_OUT3 := FALSE;
   SLAVE_28B_OUT4 := FALSE;
   SLAVE_31B_OUT1 := FALSE;
   SLAVE_31B_OUT2 := FALSE;
   SLAVE_31B_OUT3 := FALSE;
   SLAVE_31B_OUT4 := FALSE;
   SLAVE_30B_OUT1 := FALSE;
   SLAVE_30B_OUT2 := FALSE;
   SLAVE_30B_OUT3 := FALSE;
   SLAVE_30B_OUT4 := FALSE;
END_DATA_BLOCK

